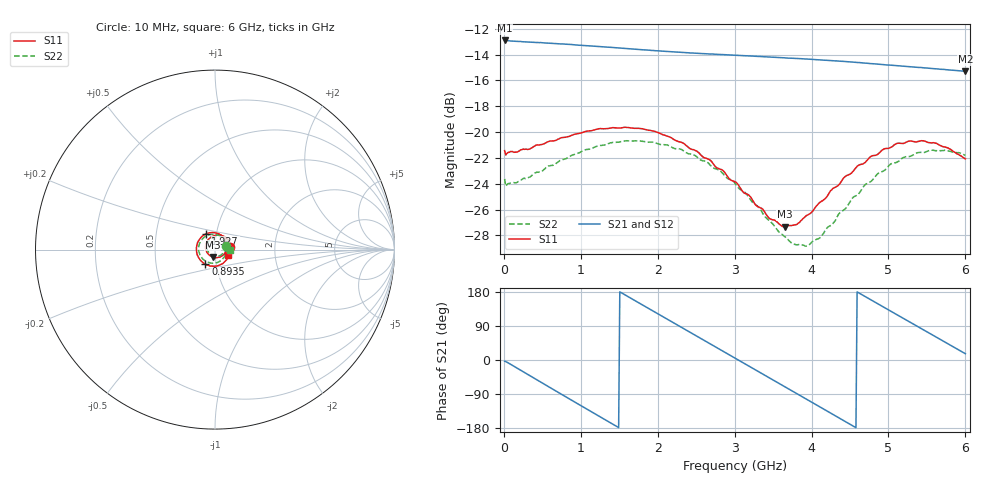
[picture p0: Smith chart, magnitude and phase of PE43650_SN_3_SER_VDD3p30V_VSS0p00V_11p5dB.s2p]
!Keysight Technologies,N5245B,MY57181451,A.13.50.07
!Date: Tuesday, May 07, 2019 08:00:08
!Correction: S11(Full 2 Port(1,2))
!S21(Full 2 Port(1,2))
!S12(Full 2 Port(1,2))
!S22(Full 2 Port(1,2))
!S2P File: Measurements: S11, S21, S12, S22:
# Hz S  dB  R 50
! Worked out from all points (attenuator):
!   401 points, 10 MHz to 6 GHz, reference 50 ohm
!   highest |S21| = -12.90 dB at 10 MHz (marker M1); lowest = -15.3 dB at 6 GHz (marker M2)
!   lowest |S11| = -27.3 dB at 3.649 GHz (marker M3), VSWR 1.09, Z = 48.5 - j3.98 ohm
!   |S11| at or under -10 dB: start of sweep to end of sweep
!   |S22| runs from -28.8 to -20.7 dB; largest |S21 - S12| = 0.0017
!   S11 on the Smith chart (normalised r, x): 10 MHz: 1.18, +0.04; 893.5 MHz: 0.89, -0.15; 1.927 GHz: 0.89, +0.16; 6 GHz: 1.15, -0.07
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1e7  -21.44 10.6  -12.90 -3.4  -12.96 -3.4  -23.62 16.0
2.496e8  -21.31 -36.9  -13.00 -30.7  -13.05 -30.7  -23.60 -36.3
5.04175e8  -20.94 -72.6  -13.08 -61.2  -13.13 -61.2  -23.00 -72.2
8.93525e8  -20.22 -123.1  -13.23 -107.6  -13.28 -107.6  -21.77 -121.0
1.013325e9  -20.05 -137.7  -13.28 -121.8  -13.33 -121.8  -21.49 -135.0
1.462575e9  -19.67 170.9  -13.46 -174.8  -13.53 -174.8  -20.79 176.7
1.6872e9  -19.70 146.0  -13.57 158.7  -13.63 158.7  -20.69 153.7
1.9268e9  -19.90 120.3  -13.67 130.7  -13.73 130.7  -20.77 129.6
2.01665e9  -20.07 110.9  -13.71 120.2  -13.76 120.2  -20.92 120.9
2.241275e9  -20.67 86.6  -13.80 94.0  -13.85 94.1  -21.28 98.4
2.4659e9  -21.36 61.5  -13.88 67.9  -13.93 67.9  -21.75 76.0
2.750425e9  -22.68 29.5  -13.97 34.7  -14.02 34.8  -22.85 46.3
3.005e9  -23.84 -3.4  -14.04 5.1  -14.10 5.2  -23.96 18.5
3.3045e9  -25.78 -47.2  -14.13 -29.9  -14.18 -29.8  -25.78 -19.8
3.648925e9  -27.33 -108.0  -14.24 -70.1  -14.29 -70.0  -28.08 -72.9
3.7837e9  -27.19 -133.3  -14.28 -85.8  -14.33 -85.8  -28.69 -97.8
4.008325e9  -26.17 -173.2  -14.37 -112.1  -14.41 -112.0  -28.49 -140.8
4.517475e9  -23.18 116.0  -14.57 -171.6  -14.62 -171.5  -25.23 139.3
4.757075e9  -21.95 88.8  -14.69 160.4  -14.74 160.6  -23.87 111.7
5.01165e9  -21.23 62.9  -14.81 130.9  -14.86 131.1  -22.56 83.9
5.475875e9  -20.71 19.7  -15.02 77.1  -15.08 77.2  -21.56 40.4
6e9  -22.08 -22.5  -15.29 16.6  -15.34 16.6  -21.81 -2.3
